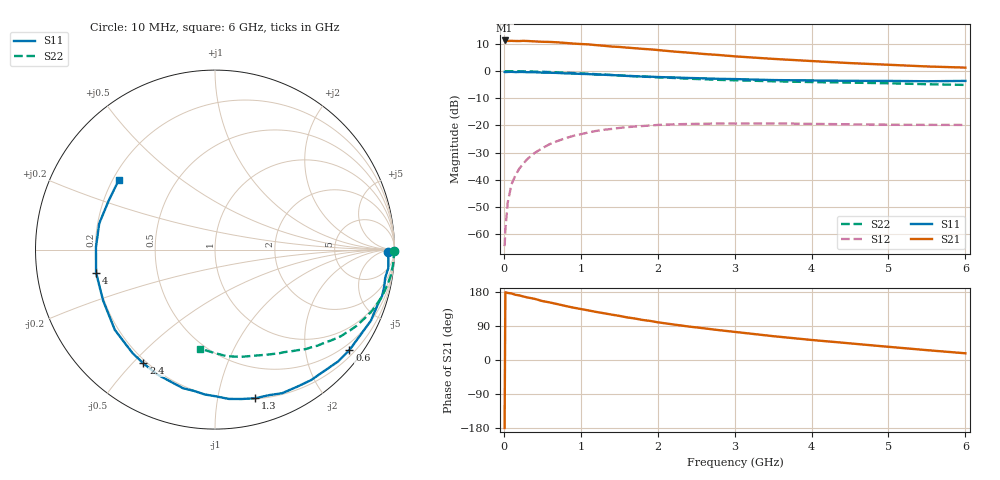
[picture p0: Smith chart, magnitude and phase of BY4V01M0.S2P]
! SIEMENS Small Signal Semiconductors
! BFY420
! Si NPN RF SIEGET Grounded Emitter Transistor in MICRO-X
! VCE = 4 V  IC = 1 mA
! Common Emitter S-Parameters:  October  1996
# GHz  S  MA  R  50
!  f  S11  S21  S12  S22
! GHz  MAG  ANG  MAG  ANG  MAG  ANG  MAG  ANG
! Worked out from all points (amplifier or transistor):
!   36 points, 10 MHz to 6 GHz, reference 50 ohm
!   highest |S21| = 11.3 dB at 10 MHz (marker M1)
!   |S21| within 3 dB of that: start of sweep to 1.763 GHz
!   unconditionally stable (mu >= 1): 4.468 GHz to end of sweep
!   at 250 MHz: K = 0.04, MSG = 22.7 dB, |S12| = -34.2 dB
!   at 1.4 GHz: K = 0.18, MSG = 15.2 dB, |S12| = -21.3 dB
!   at 6 GHz: K = 1.35, MAG = 7.0 dB, |S12| = -19.8 dB
!   S11 on the Smith chart (normalised r, x): 10 MHz: 50, -20; 600 MHz: 0.33, -2.97; 1.3 GHz: 0.20, -1.29; 2.4 GHz: 0.19, -0.54; 4 GHz: 0.20, -0.09; 6 GHz: 0.22, +0.31
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0.01  0.9662 -0.8  3.673 -179.4  0.0006 77.8  0.9989 -0.3
0.02  0.9619 -1.1  3.661 178.8  0.0012 74.6  0.9917 -0.5
0.05  0.9675 -3.2  3.598 177.0  0.0038 86.7  0.9978 -1.4
0.1  0.9708 -6.2  3.612 175.6  0.0083 82.9  0.9961 -2.8
0.15  0.9611 -9.3  3.589 172.1  0.012 82.6  0.9957 -4.2
0.2  0.9652 -12.4  3.582 170.5  0.016 83.1  0.9944 -5.5
0.3  0.9575 -18.4  3.594 165.3  0.0237 78.9  0.9901 -8.3
0.4  0.9545 -24.5  3.528 161.4  0.0312 74.9  0.9819 -11.0
0.5  0.9395 -30.6  3.473 155.6  0.0382 71.7  0.9735 -13.6
0.6  0.935 -36.8  3.449 151.8  0.0456 68.5  0.963 -16.3
0.8  0.9098 -48.0  3.306 142.7  0.0582 61.1  0.9383 -21.4
1.1  0.8832 -64.9  3.112 130.8  0.0745 52.0  0.8955 -28.3
1.3  0.8582 -74.8  2.933 123.4  0.0833 46.3  0.8652 -32.4
1.8  0.7956 -98.7  2.575 105.8  0.0976 34.2  0.794 -41.4
2.2  0.7662 -115.0  2.301 93.9  0.1049 26.4  0.7499 -47.7
2.4  0.749 -122.2  2.19 88.4  0.1066 23.3  0.7253 -50.6
2.8  0.7211 -135.3  1.98 78.7  0.1086 17.5  0.6903 -55.8
3.5  0.6849 -155.6  1.683 62.9  0.1091 10.5  0.6512 -64.1
4  0.6751 -169.0  1.535 52.9  0.1071 7.3  0.6292 -70.1
4.5  0.6633 178.8  1.407 43.9  0.1051 5.0  0.6147 -76.4
5.5  0.652 155.4  1.22 26.0  0.1026 4.5  0.5749 -90.7
6  0.6612 144.3  1.162 17.7  0.1024 5.7  0.5576 -98.8
